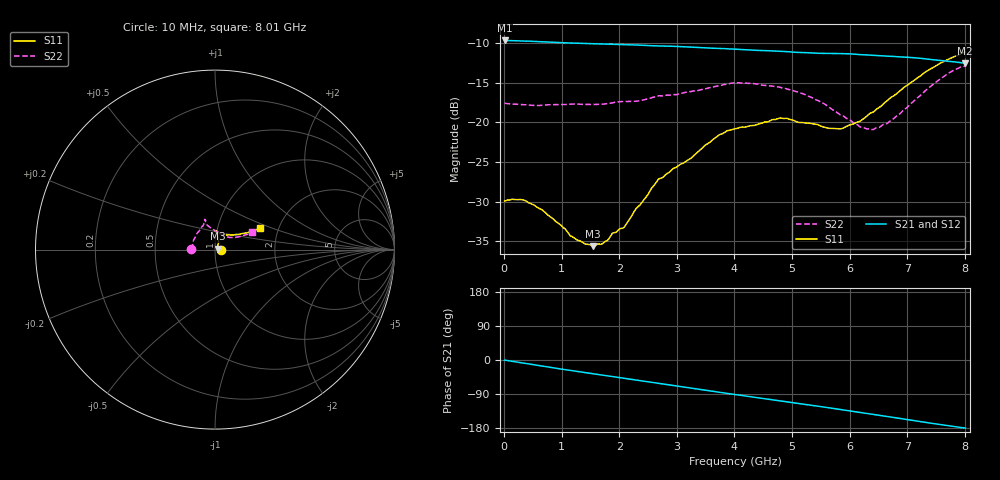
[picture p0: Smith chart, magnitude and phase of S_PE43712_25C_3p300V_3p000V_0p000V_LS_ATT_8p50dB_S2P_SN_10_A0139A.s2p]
! DEVICE ID: PE43712
! File Path: z:\PE43713\PE43713_CHAR_NOM_04292014\AMB\3p300\LS_ATT_8p50dB\PE43713_AMB_3p300V_3p000V_0p000V_LS_ATT_8p50dB_S2P_SN_10_A0139A.s2p
! Serial: 10
! Lot: A0139A
! Temp: 25C
! VDD: 3.300
! VSS: 0.000
! Control_Hi: 3.000
! Control_Lo: 0.000
! Attenuation Step: 8.50dB
! Port 1: RF1
! Port 2: RF2
! ThroughPath:1-2
! IDD: 0.0001466494
! ISS: -8.72e-008
#  Hz  S  RI  R  50
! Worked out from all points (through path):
!   801 points, 10 MHz to 8.01 GHz, reference 50 ohm
!   highest |S21| = -9.66 dB at 10 MHz (marker M1); lowest = -12.5 dB at 8 GHz (marker M2)
!   group delay of S21, straight-line fit = 61.7 ps
!   lowest |S11| = -35.6 dB at 1.55 GHz (marker M3), VSWR 1.03, Z = 51.6 + j0.443 ohm
!   |S11| at or under -10 dB: start of sweep to end of sweep
!   |S22| runs from -20.9 to -12.9 dB; largest |S21 - S12| = 0.0011
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1e7  0.0319 0.000122  0.3288 -0.00183  0.3288 -0.00177  -0.1323 0.000869
3e8  0.0324 -0.00375  0.3237 -0.0433  0.3236 -0.0433  -0.1288 0.014
5e8  0.03 -0.00509  0.3168 -0.0701  0.3169 -0.07  -0.1263 0.0222
9.6e8  0.0226 -0.00371  0.2934 -0.1257  0.2935 -0.1258  -0.1221 0.043
1.17e9  0.0191 -0.00137  0.2799 -0.1481  0.28 -0.1483  -0.1193 0.0526
1.35e9  0.0176 0.000652  0.2676 -0.1666  0.2677 -0.1667  -0.1157 0.0596
1.55e9  0.016 0.00429  0.2524 -0.1859  0.2525 -0.1859  -0.1096 0.0693
1.72e9  0.0153 0.00803  0.2387 -0.2012  0.2387 -0.2012  -0.1054 0.0767
2.09e9  0.0143 0.0167  0.2054 -0.2313  0.2055 -0.2312  -0.0975 0.0939
2.68e9  0.0197 0.0391  0.1448 -0.2669  0.1448 -0.2669  -0.0732 0.1276
3.24e9  0.016 0.0571  0.0817 -0.2871  0.0817 -0.2872  -0.0612 0.1441
3.72e9  0.014 0.0814  0.0272 -0.2917  0.027 -0.2916  -0.0559 0.1608
4.01e9  0.0104 0.0907  -0.00559 -0.2898  -0.00563 -0.2897  -0.0583 0.1676
4.79e9  0.00505 0.1064  -0.087 -0.2672  -0.0871 -0.2674  -0.0537 0.1577
5.35e9  0.0157 0.0968  -0.1372 -0.2377  -0.1371 -0.2375  -0.0432 0.1365
5.64e9  0.0272 0.0878  -0.1604 -0.2203  -0.1602 -0.2204  -0.025 0.1222
5.88e9  0.0392 0.083  -0.1803 -0.2031  -0.1799 -0.2031  -0.00673 0.1099
6.32e9  0.0757 0.0817  -0.2085 -0.1656  -0.2081 -0.1656  0.0358 0.0837
6.68e9  0.1127 0.0832  -0.2258 -0.1317  -0.2255 -0.1318  0.0731 0.069
7.55e9  0.21 0.1022  -0.2423 -0.0432  -0.2421 -0.0433  0.1671 0.081
8e9  0.2494 0.1203  -0.2363 -0.00274  -0.2362 -0.00304  0.2045 0.096
8.01e9  0.2501 0.1211  -0.2363 -0.00213  -0.2361 -0.00241  0.2051 0.0962
